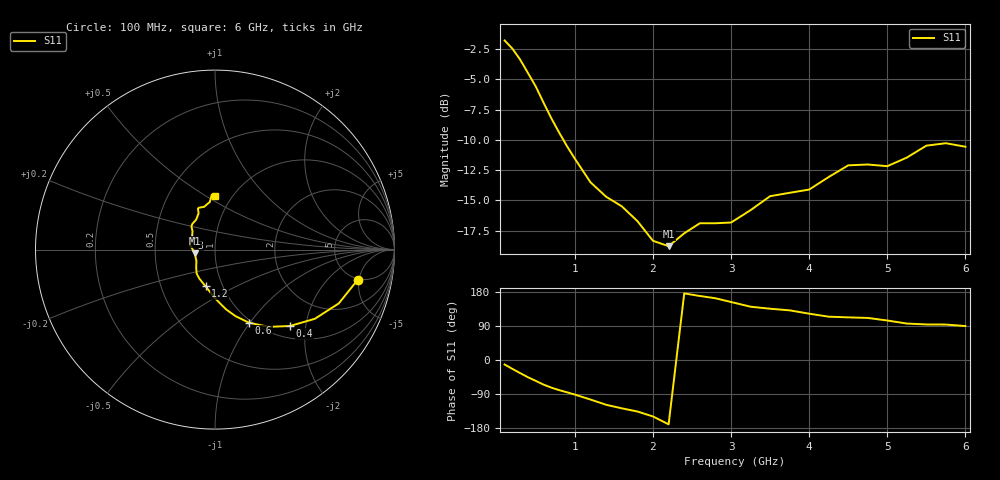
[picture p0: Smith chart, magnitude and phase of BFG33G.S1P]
! Filename:  BFG33G.S1P  Version:  2.0
! Philips part #: BFG 33  Date: Jul 1990
! Bias condition: Vce=5V, Ic=10mA
! IN LINE PINNING: same data as with cross emitter pinning.
! S1P
#  MHz  S  MA  R  50
! Freq  S11
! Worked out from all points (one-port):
!   32 points, 100 MHz to 6 GHz, reference 50 ohm
!   lowest |S11| = -18.8 dB at 2.2 GHz (marker M1), VSWR 1.26, Z = 39.8 - j1.64 ohm
!   |S11| at or under -10 dB: 851.5 MHz to end of sweep
!   S11 on the Smith chart (normalised r, x): 100 MHz: 4.85, -4.80; 400 MHz: 1.24, -1.63; 600 MHz: 0.97, -0.99; 1.2 GHz: 0.83, -0.36; 3 GHz: 0.77, +0.10; 6 GHz: 0.84, +0.55
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100  0.813 -11.9
200  0.752 -23.5
300  0.677 -34.7
400  0.596 -45.6
500  0.524 -55.2
600  0.449 -65.1
700  0.387 -73.0
900  0.297 -85.3
1200  0.211 -104.4
1400  0.184 -118.2
1600  0.168 -127.5
1800  0.146 -135.9
2000  0.121 -149.0
2200  0.115 -169.8
2400  0.13 175.8
2600  0.143 168.9
3000  0.144 153.0
3250  0.162 140.6
3500  0.185 135.3
4000  0.197 122.2
4250  0.222 114.3
4500  0.248 112.5
4750  0.25 111.0
5000  0.246 104.2
5250  0.267 96.2
5500  0.299 93.8
5750  0.306 93.5
6000  0.296 89.6
